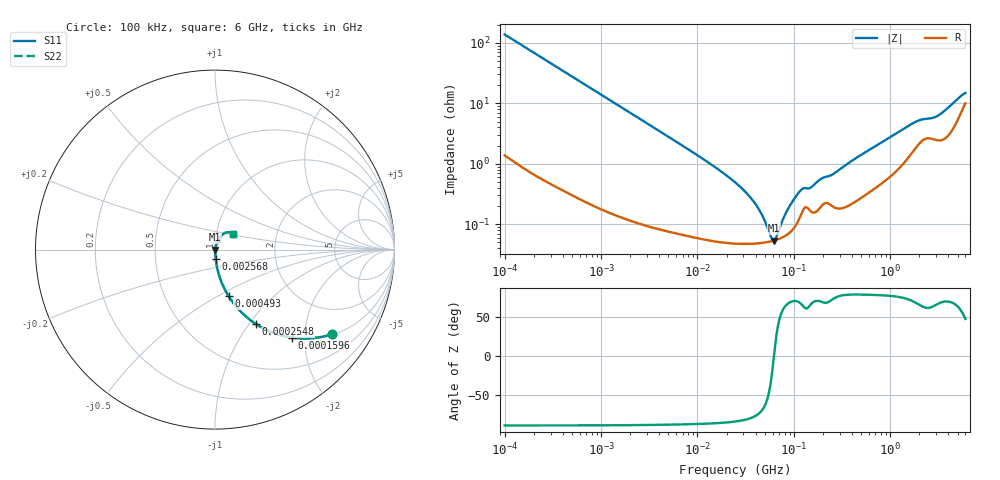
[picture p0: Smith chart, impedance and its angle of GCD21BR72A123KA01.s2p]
!Murata Part Number: GCD21BR72A123KA01
!These Parameters are Measured in Series Mode Connection
!Data Generated on Jan 08, 2026
!  o--ll--o
!Port1  Port2
!  o------o
!Operation Temp=25[degC], DC Bias Voltage=0[V]
!Freq. Start=100[kHz] Stop=6[GHz] 401[Steps]
# Hz S RI R 50
!Freq.(Hz) S11(Real) S11(Imag) S21(Real) S21(Imag) S12(Real) S12(Imag) S22(Real) S22(Imag)
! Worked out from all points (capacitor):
!   401 points, 100 kHz to 6 GHz, reference 50 ohm
!   read as one part in series: C = 11.6 nF near 105.7 kHz
!   lowest |Z| = 53.9 mohm at 62.4 MHz (marker M1)
!   series resonance near 62.06 MHz, so ESL is about 570 pH
!   S11 on the Smith chart (normalised r, x): 100 kHz: 1.03, -2.75; 159.6 kHz: 1.02, -1.73; 254.8 kHz: 1.01, -1.08; 493 kHz: 1.01, -0.56; 2.568 MHz: 1.00, -0.11; 6 GHz: 1.20, +0.22
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100000  0.6524 -0.4712  0.3476 0.4712  0.3476 0.4712  0.6524 -0.4712
159614  0.4279 -0.49  0.5721 0.49  0.5721 0.49  0.4279 -0.49
254767  0.2295 -0.4156  0.7705 0.4156  0.7705 0.4156  0.2295 -0.4156
492983  0.0757 -0.2592  0.9243 0.2592  0.9243 0.2592  0.0757 -0.2592
631452  0.0483 -0.2088  0.9517 0.2088  0.9517 0.2088  0.0483 -0.2088
2567761  0.00395 -0.0542  0.996 0.0542  0.996 0.0542  0.00395 -0.0542
3987316  0.00205 -0.035  0.9979 0.035  0.9979 0.035  0.00205 -0.035
1.337449e7  0.00064 -0.0101  0.9994 0.0101  0.9994 0.0101  0.00064 -0.0101
2.517799e7  0.0005 -0.00474  0.9995 0.00474  0.9995 0.00474  0.0005 -0.00474
4.018763e7  0.000484 -0.00208  0.9995 0.00208  0.9995 0.00208  0.000484 -0.00208
4.739851e7  0.000495 -0.00127  0.9995 0.00127  0.9995 0.00127  0.000495 -0.00127
5.746221e7  0.000521 -0.00036  0.9995 0.00036  0.9995 0.00036  0.000521 -0.00036
6.240487e7  0.000538 2.66e-05  0.9995 -2.66e-05  0.9995 -2.66e-05  0.000538 2.66e-05
6.593397e7  0.000553 0.000286  0.9994 -0.000286  0.9994 -0.000286  0.000553 0.000286
8.44535e7  0.00067 0.00151  0.9993 -0.00151  0.9993 -0.00151  0.00067 0.00151
1.0524e8  0.000981 0.00274  0.999 -0.00274  0.999 -0.00274  0.000981 0.00274
1.241232e8  0.00171 0.0035  0.9983 -0.0035  0.9983 -0.0035  0.00171 0.0035
1.546735e8  0.00159 0.00391  0.9984 -0.00391  0.9984 -0.00391  0.00159 0.00391
9.76689e8  0.0066 0.026  0.9934 -0.026  0.9934 -0.026  0.0066 0.026
1.838654e9  0.0201 0.0444  0.9799 -0.0444  0.9799 -0.0444  0.0201 0.0444
3.100717e9  0.0269 0.0545  0.9731 -0.0545  0.9731 -0.0545  0.0269 0.0545
6e9  0.0997 0.0893  0.9003 -0.0893  0.9003 -0.0893  0.0997 0.0893
